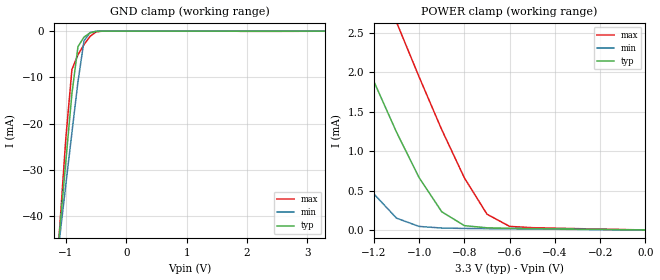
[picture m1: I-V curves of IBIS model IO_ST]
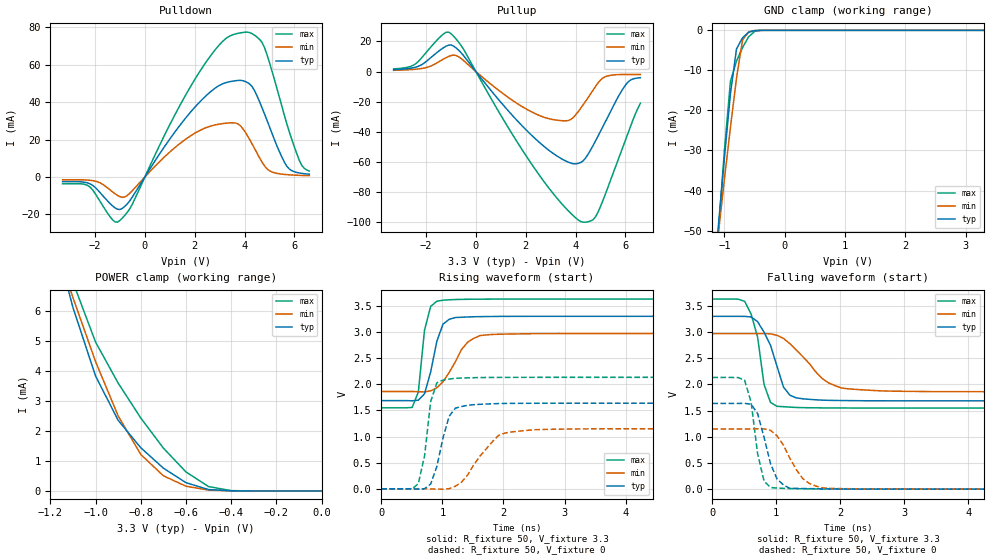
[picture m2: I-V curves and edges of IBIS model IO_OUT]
[IBIS Ver]   3.2
[Comment Char]   |_char
[File name]   sg5032can33.ibs
[File Rev]   1.0
[Date]   2015/11/24 22:00:00
[Source]
[Notes]
[Disclaimer]
This information is for modeling purposes only, and is not guaranteed.
Property of SEIKO EPSON Corp.,
unauthorized reproduction and/or distribution is strictly prohibited.
[Copyright]
Copyright 2006, SEIKO EPSON Corp.
[Component]   SG5032CAN
Si_location Pin
Timing_location Pin
[Manufacturer]   SEIKO EPSON Corp.
| COG
| COG
[Package]
R_pkg   56.75m   56.75m   56.75m
L_pkg   2.25n   2.25n   2.25n
C_pkg   0.860p   0.860p   0.860p
[Pin] signal_name   model_name
1   /ST   IO_ST
2   GND   GND
3   OUT   IO_OUT
4   Vcc   POWER
| Models and submodels in the file (2): IO_ST (Input), IO_OUT (3-state)
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[Model]   IO_ST
Model_type Input
Polarity Inverting
Vinh=2.64
Vinl=0.66
C_comp   5p   4p   6p
[Temperature Range] 25   105   -40
[Voltage Range]   3.3   2.97   3.63
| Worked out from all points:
|   GND clamp passes 1 mA (typ) near -0.67 V on its own axis
|   POWER clamp passes 1 mA (typ) near -1.06 V on its own axis
[GND Clamp]
-3.3V     -402mA     -327.9mA   -490.5mA
-1.2V     -57.55mA   -55.73mA   -61.1mA
-1.1V     -42.76mA   -44.37mA   -42.03mA
-1V       -28.06mA   -33.1mA    -23.01mA
-900mV    -13.48mA   -21.96mA   -8.307mA
-800mV    -3.366mA   -10.96mA   -5.117mA
-700mV    -1.291mA   -2.107mA   -2.916mA
-600mV    -372.7uA   -316.6uA   -1.133mA
-500mV    -50.2uA    -42.28uA   -184.2uA
-400mV    -4.138uA   -5.173uA   -10.82uA
3.3V      49.33pA    7.397uA    -16.55uA
[POWER Clamp]
-3.3V     16.34mA    14.23mA    18.13mA
-1.6V     4.626mA    2.832mA    6.156mA
-1.5V     3.937mA    2.167mA    5.452mA
-1.3V     2.559mA    945.4uA    4.043mA
-1.2V     1.883mA    457.6uA    3.339mA
-1.1V     1.241mA    150uA      2.635mA
-1V       662.9uA    44.86uA    1.939mA
-900mV    230.7uA    24.5uA     1.271mA
-800mV    54.96uA    19.51uA    660.2uA
-700mV    27.32uA    16.61uA    199.7uA
-600mV    21.62uA    14.03uA    45.16uA
0V        49.33pA    642.3pA    37.13pA
[Model]   IO_OUT
Model_type 3-state
Enable Active-High
Polarity Non-Inverting
Vmeas=1.65
C_comp   5p   4p   6p
[Temperature Range] 25   105   -40
[Voltage Range]   3.3   2.97   3.63
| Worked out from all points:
|   slope of the pulldown table from 0 to 0.495 V, typ, clamps not added: 47.8 ohm
|   slope of the pullup table from 0 to 0.495 V, typ, clamps not added: 47.8 ohm
|   GND clamp passes 1 mA (typ) near -0.64 V on its own axis
|   POWER clamp passes 1 mA (typ) near -0.74 V on its own axis
|   falling waveform, R_fixture 50, V_fixture 3.3: 20-80 % time 280ps typ, 516ps min, 182ps max; typ from 3.3 V to 1.69 V
|   falling waveform, R_fixture 50, V_fixture 0: 20-80 % time 228ps typ, 329ps min, 161ps max; typ from 1.64 V to 0 V
|   rising waveform, R_fixture 50, V_fixture 3.3: 20-80 % time 203ps typ, 343ps min, 131ps max; typ from 1.69 V to 3.3 V
|   rising waveform, R_fixture 50, V_fixture 0: 20-80 % time 212ps typ, 445ps min, 149ps max; typ from 0 V to 1.64 V
[Pullup]
-3.3V     1.222mA    818.5uA    1.762mA
-2.5V     2.555mA    1.42mA     4.276mA
-1.3V     15.85mA    8.309mA    25mA
-1V       17.67mA    10.61mA    25.22mA
-500mV    10.69mA    7.357mA    14.94mA
1.3V      -26.13mA   -17.24mA   -37.33mA
2.7V      -49.29mA   -30.2mA    -72.43mA
3.7V      -60.19mA   -32.59mA   -92.45mA
4.3V      -59.44mA   -22.2mA    -100.2mA
4.9V      -42.96mA   -7.615mA   -93.51mA
6V        -9.105mA   -1.966mA   -45.65mA
6.6V      -4.131mA   -1.97mA    -21.08mA
[Pulldown]
-3.3V     -2.505mA   -1.516mA   -3.644mA
-2.3V     -3.164mA   -1.638mA   -4.477mA
-1.3V     -15.36mA   -7.9mA     -22.77mA
-1V       -17.35mA   -10.49mA   -23.19mA
-500mV    -10.62mA   -7.231mA   -14.42mA
2.4V      42.65mA    26.02mA    60.21mA
3.6V      51.29mA    28.87mA    76.18mA
4.1V      50.51mA    22.39mA    77.3mA
4.8V      33.68mA    5.935mA    69.06mA
5.7V      5.666mA    1.251mA    28.22mA
6.2V      2.143mA    875.2uA    8.813mA
6.6V      1.49mA     707.7uA    3.165mA
[GND Clamp]
-3.3V     -485.2mA   -392.5mA   -586.9mA
-1.1V     -48.77mA   -50.63mA   -50.17mA
-1V       -31.82mA   -37.19mA   -29.98mA
-900mV    -15.78mA   -24.22mA   -12.71mA
-800mV    -4.669mA   -11.96mA   -7.684mA
-700mV    -1.852mA   -2.454mA   -4.316mA
-600mV    -505.1uA   -405.3uA   -1.654mA
-500mV    -63.64uA   -57.41uA   -272.4uA
-400mV    -4.376uA   -6.701uA   -15.57uA
3.3V      192.6pA    533.3nA    148.2pA
[POWER Clamp]
-3.3V     83.66mA    64.55mA    112.5mA
-1.2V     8.957mA    8.759mA    10.16mA
-1.1V     6.115mA    6.443mA    6.961mA
-1V       3.829mA    4.311mA    4.959mA
-900mV    2.354mA    2.501mA    3.593mA
-800mV    1.439mA    1.216mA    2.43mA
-700mV    759.3uA    504uA      1.427mA
-600mV    274.3uA    156.6uA    632.3uA
-500mV    45.05uA    27.63uA    144.7uA
-400mV    3.085uA    3.004uA    9.596uA
0V        192.4pA    826.6pA    205.6pA
[Falling Waveform]
R_fixture=50
V_fixture=3.3
V_fixture_min=2.97
V_fixture_max=3.63
0s        3.3V       2.97V      3.63V
505.1ps   3.299V     2.97V      3.587V
707.1ps   3.199V     2.971V     2.906V
808.1ps   2.997V     2.973V     1.998V
909.1ps   2.747V     2.965V     1.657V
1.01ns    2.349V     2.939V     1.582V
1.212ns   1.793V     2.778V     1.567V
1.717ns   1.699V     2.112V     1.552V
2.121ns   1.691V     1.917V     1.55V
10ns      1.687V     1.861V     1.549V
[Falling Waveform]
R_fixture=50
V_fixture=0
V_fixture_min=0
V_fixture_max=0
0s        1.637V     1.149V     2.133V
505.1ps   1.639V     1.148V     2.079V
606.1ps   1.621V     1.149V     1.66V
707.1ps   1.444V     1.152V     678.8mV
808.1ps   989.8mV    1.151V     153.5mV
909.1ps   486mV      1.123V     31.4mV
1.212ns   14.61mV    591.3mV    12.12mV
1.414ns   12.81mV    200.1mV    6.693mV
1.717ns   6.729mV    26.43mV    3.813mV
10ns      -3.836uV   -11.88uV   1.618uV
[Rising Waveform]
R_fixture=50
V_fixture=3.3
V_fixture_min=2.97
V_fixture_max=3.63
0s        1.687V     1.861V     1.549V
505.1ps   1.683V     1.862V     1.556V
606.1ps   1.695V     1.857V     1.85V
707.1ps   1.817V     1.853V     3.032V
808.1ps   2.236V     1.873V     3.49V
909.1ps   2.822V     1.933V     3.588V
1.111ns   3.242V     2.226V     3.616V
1.414ns   3.288V     2.806V     3.626V
1.717ns   3.295V     2.944V     3.629V
10ns      3.3V       2.97V      3.63V
[Rising Waveform]
R_fixture=50
V_fixture=0
V_fixture_min=0
V_fixture_max=0
0s        0V         0V         0V
606.1ps   -5.964mV   927.1uV    97.94mV
707.1ps   -174.5uV   -357.6uV   622.5mV
808.1ps   90.84mV    -3.359mV   1.668V
909.1ps   424.5mV    -6.264mV   2.027V
1.01ns    973mV      -7.605mV   2.079V
1.212ns   1.542V     48.3mV     2.114V
1.919ns   1.63V      1.02V      2.131V
2.121ns   1.634V     1.086V     2.132V
10ns      1.637V     1.149V     2.133V
[Ramp]
R_load=50
dV/dt_r   9.822E-1/2.017E-10   6.891E-1/4.373E-10   1.280E+0/1.429E-10
dV/dt_f   9.679E-1/2.740E-10   6.653E-1/5.130E-10   1.249E+0/1.784E-10
|[End   IO_OUT
